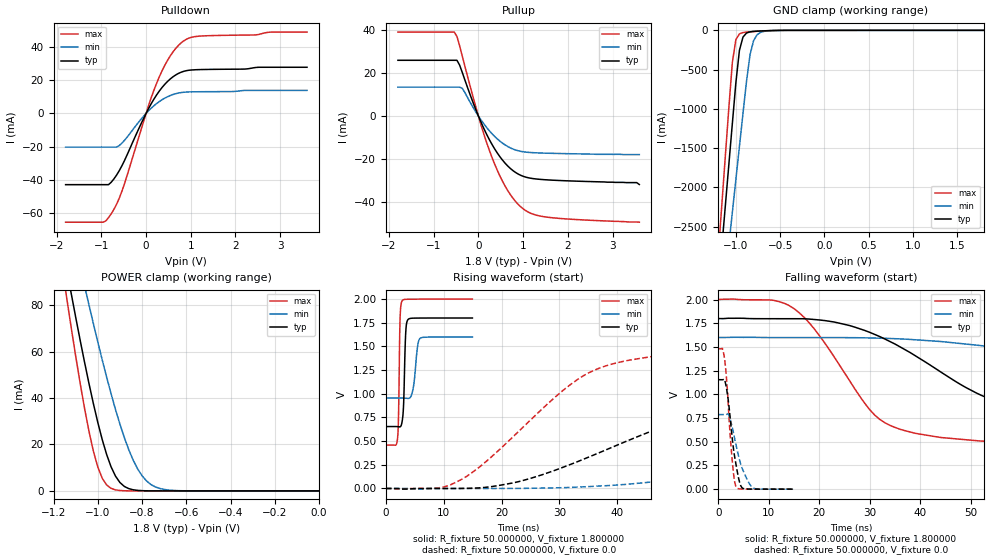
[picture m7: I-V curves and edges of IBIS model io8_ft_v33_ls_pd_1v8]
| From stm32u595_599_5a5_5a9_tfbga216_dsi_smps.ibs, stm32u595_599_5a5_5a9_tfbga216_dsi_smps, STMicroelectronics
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|   Model io8_ft_v33_ls_pd_1v8
[Model]  io8_ft_v33_ls_pd_1v8
Model_type I/O
Polarity   Non-Inverting
Enable   Active-Low
Vinl =   0.540000V
Vinh =   1.260000V
Vmeas =  0.900000V
Cref =   50.000000pF
Rref =   100.000000M
Vref =   0.0V
C_comp   3.087500pF   3.086600pF   3.135700pF
[Temperature Range]   25.000000   0.140000k   -40.000000
[Pullup Reference]   1.800000V   1.600000V   2.000000V
[Pulldown Reference]   0.0V   0.0V   0.0V
[POWER Clamp Reference]   1.800000V   1.600000V   2.000000V
[GND Clamp Reference]   0.0V   0.0V   0.0V
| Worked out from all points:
|   slope of the pulldown table from 0 to 0.27 V, typ, clamps not added: 21.7 ohm
|   slope of the pullup table from 0 to 0.27 V, typ, clamps not added: 22.6 ohm
|   GND clamp passes 1 mA (typ) near -0.51 V on its own axis
|   POWER clamp passes 1 mA (typ) near -0.86 V on its own axis
|   rising waveform, R_fixture 50.000000, V_fixture 1.800000: 20-80 % time 315ps typ, 629ps min, 226ps max; typ from 0.654 V to 1.8 V
|   rising waveform, R_fixture 50.000000, V_fixture 0.0: 20-80 % time 31.3ns typ, 66.8ns min, 16.4ns max; typ from 0 V to 1.15 V
|   falling waveform, R_fixture 50.000000, V_fixture 1.800000: 20-80 % time 24.6ns typ, 55.5ns min, 12.3ns max; typ from 1.8 V to 0.654 V
|   falling waveform, R_fixture 50.000000, V_fixture 0.0: 20-80 % time 1.6ns typ, 2.38ns min, 1.17ns max; typ from 1.15 V to 0 V
[Pulldown]
|Voltage   I(typ)   I(min)   I(max)
-1.8V     -42.74mA   -20.21mA   -65.25mA
-960mV    -42.74mA   -20.21mA   -65.25mA
-780mV    -41.3mA    -20.21mA   -60.25mA
-660mV    -37mA      -20.2mA    -54.5mA
-540mV    -31.39mA   -17.82mA   -46.65mA
0V        0A         0A         0A
240mV     11.28mA    6.002mA    18.38mA
480mV     19.17mA    10.02mA    31.83mA
780mV     24.67mA    12.5mA     42.21mA
960mV     25.9mA     12.9mA     45.21mA
1.14V     26.24mA    12.99mA    46.23mA
3.6V      27.69mA    13.82mA    48.79mA
[Pullup]
|Voltage   I(typ)   I(min)   I(max)
-1.8V     26.06mA    13.5mA     39.23mA
-540mV    26.06mA    13.5mA     39.23mA
-480mV    26.06mA    13.5mA     37.19mA
-360mV    20.34mA    12.93mA    27.94mA
0V        0A         0A         0A
300mV     -13.1mA    -8.158mA   -19.11mA
480mV     -18.98mA   -11.71mA   -27.97mA
660mV     -23.42mA   -14.29mA   -34.95mA
1.02V     -28.29mA   -16.75mA   -43.65mA
1.26V     -29.33mA   -17.15mA   -46.11mA
1.62V     -29.92mA   -17.41mA   -47.45mA
3.6V      -32mA      -18mA      -49.6mA
[GND_clamp]
|Voltage   I(typ)   I(min)   I(max)
-1.8V     -9.707A    -9.942A    -9.774A
-1.2V     -3.309A    -4.006A    -2.865A
-1.16V    -2.777A    -3.584A    -2.239A
-1.12V    -2.246A    -3.162A    -1.614A
-1.04V    -1.186A    -2.319A    -408.7mA
-1V       -663.9mA   -1.898A    -117.8mA
-960mV    -254mA     -1.478A    -45.15mA
-920mV    -86.04mA   -1.06A     -28.6mA
-840mV    -19.13mA   -308.9mA   -18.75mA
-800mV    -13.4mA    -130.8mA   -15.33mA
-720mV    -7.959mA   -25.38mA   -9.395mA
1.8V      45.71uA    33.33uA    56.11uA
[POWER_clamp]
|Voltage   I(typ)   I(min)   I(max)
-1.8V     470.8mA    433.7mA    554.6mA
-1.14V    95.25mA    122.7mA    82.82mA
-1.12V    84.97mA    114mA      70.27mA
-1.06V    55.51mA    88.42mA    35.67mA
-1.04V    46.34mA    80.15mA    25.76mA
-1V       29.51mA    64.13mA    10.3mA
-940mV    10.39mA    41.86mA    1.109mA
-900mV    3.624mA    28.77mA    182.8uA
-840mV    490.7uA    13.24mA    11.35uA
-800mV    116.8uA    6.532mA    1.77uA
-740mV    13.2uA     1.723mA    109.3nA
0V        0A         18.72nA    0A
[Ramp]
| variable   typ   min   max
dV/dt_r  0.69258/31.26758n   0.47164/66.70023n   0.88830/16.41237n
dV/dt_f  0.68753/24.57660n   0.38695/55.42667n   0.92452/12.27350n
R_load = 50.000000
[Rising Waveform]
R_fixture= 50.000000
V_fixture= 1.800000
V_fixture_min= 1.600000
V_fixture_max= 2.000000
|time   V(typ)   V(min)   V(max)
0s        653.5mV    954.4mV    458.4mV
2.012ns   653mV      954.5mV    524.2mV
2.192ns   651.7mV    954.5mV    777mV
2.462ns   651.2mV    954.5mV    1.801V
2.793ns   700.2mV    954.4mV    1.979V
3.063ns   884.6mV    954.2mV    1.993V
3.423ns   1.635V     953.1mV    1.997V
3.754ns   1.777V     950.9mV    1.997V
5.856ns   1.799V     1.581V     1.998V
14.95ns   1.799V     1.599V     1.999V
[Rising Waveform]
R_fixture= 50.000000
V_fixture= 0.0
V_fixture_min= 0.0
V_fixture_max= 0.0
|time   V(typ)   V(min)   V(max)
0s        2.158nV    142.4nV    1.475nV
13.01ns   773.9uV    -136.1uV   93.54mV
23.02ns   73.55mV    888.6uV    606.9mV
31.03ns   233.7mV    9.42mV     1.056V
37.04ns   381.8mV    26.18mV    1.274V
58.06ns   859.6mV    157.9mV    1.448V
87.09ns   1.096V     403.3mV    1.477V
120.1ns   1.141V     609.8mV    1.48V
166.2ns   1.153V     735.3mV    1.48V
498.5ns   1.154V     786.2mV    1.48V
[Falling Waveform]
R_fixture= 50.000000
V_fixture= 1.800000
V_fixture_min= 1.600000
V_fixture_max= 2.000000
|time   V(typ)   V(min)   V(max)
0s        1.799V     1.599V     1.999V
11.01ns   1.798V     1.599V     1.991V
15.02ns   1.798V     1.598V     1.904V
20.02ns   1.785V     1.598V     1.622V
30.03ns   1.654V     1.595V     837.7mV
33.03ns   1.583V     1.591V     700.1mV
52.05ns   991.5mV    1.514V     507.6mV
79.08ns   735.3mV    1.278V     468.3mV
143.1ns   660.8mV    1.02V      458.7mV
498.5ns   653.5mV    954.4mV    458.4mV
[Falling Waveform]
R_fixture= 50.000000
V_fixture= 0.0
V_fixture_min= 0.0
V_fixture_max= 0.0
|time   V(typ)   V(min)   V(max)
0s        1.154V     786.2mV    1.48V
840.8ps   1.154V     786.2mV    1.481V
1.291ns   1.149V     786mV      1.363V
1.982ns   943.1mV    791.1mV    902.4mV
2.763ns   546.9mV    656.1mV    312.9mV
3.153ns   378.1mV    560.7mV    114.4mV
3.514ns   264.7mV    471mV      27.18mV
4.685ns   17.23mV    228.6mV    1.213mV
6.637ns   667uV      24.29mV    -120.2uV
14.95ns   2.158nV    142.4nV    1.475nV
